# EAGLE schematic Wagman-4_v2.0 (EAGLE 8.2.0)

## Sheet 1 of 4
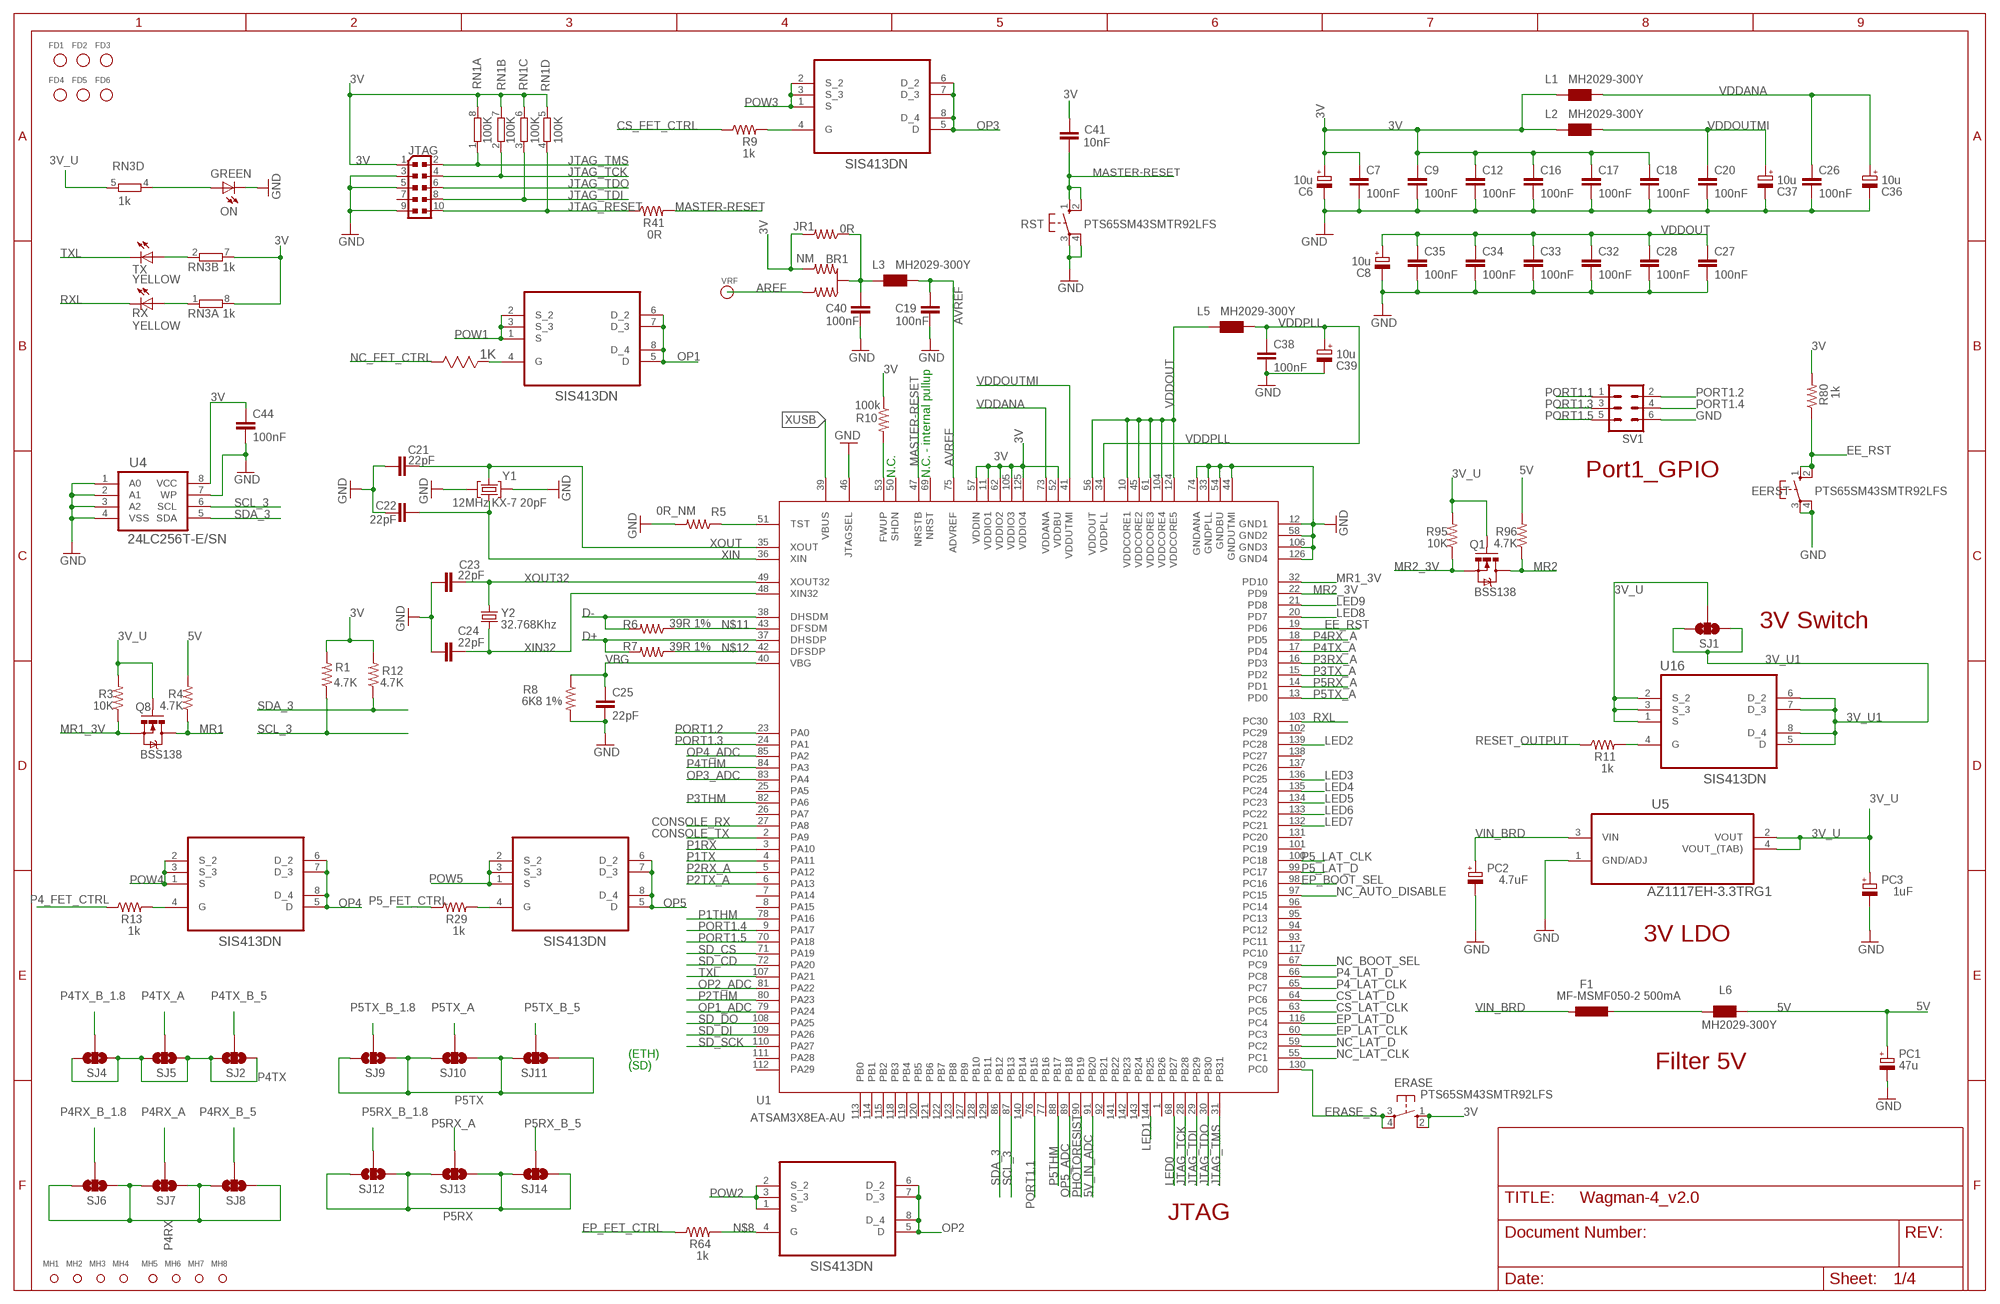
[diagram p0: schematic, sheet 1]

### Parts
BR1  NM  J0402  [J0402]
C6  10u  CPOL-EUSMCB  [SMC_B]
C7  100nF  CAP0805  [0805]
C8  10u  CPOL-EUSMCB  [SMC_B]
C9  100nF  CAP0805  [0805]
C12  100nF  CAP0805  [0805]
C16  100nF  CAP0805  [0805]
C17  100nF  CAP0805  [0805]
C18  100nF  CAP0805  [0805]
C19  100nF  CAP0805  [0805]
C20  100nF  CAP0805  [0805]
C21  22pF  CAP0805  [0805]
C22  22pF  CAP0805  [0805]
C23  22pF  CAP0805  [0805]
C24  22pF  CAP0805  [0805]
C25  22pF  CAP0805  [0805]
C26  100nF  CAP0805  [0805]
C27  100nF  CAP0805  [0805]
C28  100nF  CAP0805  [0805]
C32  100nF  CAP0805  [0805]
C33  100nF  CAP0805  [0805]
C34  100nF  CAP0805  [0805]
C35  100nF  CAP0805  [0805]
C36  10u  CPOL-EUSMCB  [SMC_B]
C37  10u  CPOL-EUSMCB  [SMC_B]
C38  100nF  CAP0805  [0805]
C39  10u  CPOL-EUSMCB  [SMC_B]
C40  100nF  CAP0805  [0805]
C41  10nF  CAP0805  [0805]
C44  100nF  CAP0805  [0805]
EERST  PTS65SM43SMTR92LFS  [TACT_SPST_SMD_6X6]
ERASE  PTS65SM43SMTR92LFS  [TACT_SPST_SMD_6X6]
F1  MF-MSMF050-2 500mA  L-EUL1812  [L1812]
FD1  FIDUCIAL-1MM  [FD-1MM]
FD2  FIDUCIAL-1MM  [FD-1MM]
FD3  FIDUCIAL-1MM  [FD-1MM]
FD4  FIDUCIAL-1MM  [FD-1MM]
FD5  FIDUCIAL-1MM  [FD-1MM]
FD6  FIDUCIAL-1MM  [FD-1MM]
JR1  0R  RESISTOR0805-RES  [0805]
JTAG  PINHEAD_PINHD-2X5PASSO127  [PINHEAD_2X05_127]
L1  MH2029-300Y  WE-CBF_0805  [0805]
L2  MH2029-300Y  WE-CBF_0805  [0805]
L3  MH2029-300Y  WE-CBF_0805  [0805]
L5  MH2029-300Y  WE-CBF_0805  [0805]
L6  MH2029-300Y  WE-CBF_0805  [0805]
MH1  MH-3.964  [MH3.964]
MH2  MH-3.964  [MH3.964]
MH3  MH-3.964  [MH3.964]
MH4  MH-3.964  [MH3.964]
MH5  MH-3.964  [MH3.964]
MH6  MH-3.964  [MH3.964]
MH7  MH-3.964  [MH3.964]
MH8  MH-3.964  [MH3.964]
ON  GREEN  LEDCHIPLED_0805  [CHIPLED_0805]
PC1  47u  CPOL-EUD  [PANASONIC_D]
PC2  4.7uF  CPOL-EUD  [PANASONIC_D]
PC3  1uF  CPOL-EUD  [PANASONIC_D]
Q1  BSS138  MOSFET-NCHANNELSMD  [SOT23-3]
Q8  BSS138  MOSFET-NCHANNELSMD  [SOT23-3]
R1  4.7K  RESISTOR0805-RES  [0805]
R3  10K  RESISTOR0805-RES  [0805]
R4  4.7K  RESISTOR0805-RES  [0805]
R5  0R_NM  RESISTOR0805-RES  [0805]
R6  39R 1%  RESISTOR0805-RES  [0805]
R7  39R 1%  RESISTOR0805-RES  [0805]
R8  6K8 1%  RESISTOR0805-RES  [0805]
R9  1k  RESISTOR0805-RES  [0805]
R10  100k  RESISTOR0805-RES  [0805]
R11  1k  RESISTOR0805-RES  [0805]
R12  4.7K  RESISTOR0805-RES  [0805]
R13  1k  RESISTOR0805-RES  [0805]
R29  1k  RESISTOR0805-RES  [0805]
R30  1K  CRM0805-FW-R050ELF  [0805]
R41  0R  RESISTOR0805-RES  [0805]
R64  1k  RESISTOR0805-RES  [0805]
R80  1k  RESISTOR0805-RES  [0805]
R95  10K  RESISTOR0805-RES  [0805]
R96  4.7K  RESISTOR0805-RES  [0805]
RN1  100K  4R-NCAT16  [CAT16]
RN3  1k  4R-NCAT16  [CAT16]
RST  PTS65SM43SMTR92LFS  [TACT_SPST_SMD_6X6]
RX  YELLOW  LEDCHIPLED_0805  [CHIPLED_0805]
SJ1  SOLDERJUMPER_2WAYPASTE1&2&3  [SJ_3_PASTE1&2&3]
SJ2  SOLDERJUMPER_2WAYPASTE1&2&3  [SJ_3_PASTE1&2&3]
SJ4  SOLDERJUMPER_2WAYPASTE1&2&3  [SJ_3_PASTE1&2&3]
SJ5  SOLDERJUMPER_2WAYPASTE1&2&3  [SJ_3_PASTE1&2&3]
SJ6  SOLDERJUMPER_2WAYPASTE1&2&3  [SJ_3_PASTE1&2&3]
SJ7  SOLDERJUMPER_2WAYPASTE1&2&3  [SJ_3_PASTE1&2&3]
SJ8  SOLDERJUMPER_2WAYPASTE1&2&3  [SJ_3_PASTE1&2&3]
SJ9  SOLDERJUMPER_2WAYPASTE1&2&3  [SJ_3_PASTE1&2&3]
SJ10  SOLDERJUMPER_2WAYPASTE1&2&3  [SJ_3_PASTE1&2&3]
SJ11  SOLDERJUMPER_2WAYPASTE1&2&3  [SJ_3_PASTE1&2&3]
SJ12  SOLDERJUMPER_2WAYPASTE1&2&3  [SJ_3_PASTE1&2&3]
SJ13  SOLDERJUMPER_2WAYPASTE1&2&3  [SJ_3_PASTE1&2&3]
SJ14  SOLDERJUMPER_2WAYPASTE1&2&3  [SJ_3_PASTE1&2&3]
SV1  MA03-2  [MA03-2]
TX  YELLOW  LEDCHIPLED_0805  [CHIPLED_0805]
U1  ATSAM3X8EA-AU  ATSAM3X/AAU  [LQFP144]
U3  SIS413DN  [SIS413]
U4  24LC256T-E/SN  [SOIC8]
U5  AZ1117EH-3.3TRG1  [SOT230P700X180-4N]
U6  SIS413DN  [SIS413]
U7  SIS413DN  [SIS413]
U8  SIS413DN  [SIS413]
U9  SIS413DN  [SIS413]
U16  SIS413DN  [SIS413]
VRF  FIDUCIAL-1MM  [FD-1MM]
Y1  12MHz KX-7 20pF  CRYSTAL-3.2-2.5  [CRYSTAL-3.2-2.5]
Y2  32.768Khz  RESONATOR_EPSON_FC_145  [RESONATOR_EPSON_FC_145]

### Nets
3V: BR1.3 C6.+ C7.1 C9.1 C12.1 C16.1 C17.1 C18.1 C41.1 C44.1 ERASE.1 ERASE.2 JR1.2 JTAG.1 L1.1 L2.1 R1.2 R10.1 R12.2 R80.2 RN1.5 RN1.6 RN1.7 RN1.8 RN3.7 RN3.8 U1.11(VDDIO1) U1.52(VDDBU) U1.57(VDDIN) U1.62(VDDIO2) U1.105(VDDIO3) U1.125(VDDIO4) U4.8(VCC) ; also sheet 2,3,4
3V_U: PC3.+ Q1.1(G) Q8.1(G) R3.2 R95.2 RN3.5 SJ1.2 U5.2(VOUT) U5.4(VOUT_(TAB)) U16.1(S) U16.2(S_2) U16.3(S_3) ; also sheet 2,3,4
3V_U1: SJ1.1 SJ1.3 U16.5(D) U16.6(D_2) U16.7(D_3) U16.8(D_4) ; also sheet 3
5V: L6.1 PC1.+ R4.2 R96.2 ; also sheet 2,3,4
5V_IN_ADC: U1.91(PB20) ; also sheet 4
AREF: BR1.1 VRF.1
AVREF: C19.1 L3.2 U1.75(ADVREF)
AVREFL: BR1.2(C) C40.1 JR1.1 L3.1
CONSOLE_RX: U1.27(PA8) ; also sheet 4
CONSOLE_TX: U1.2(PA9) ; also sheet 4
CS_FET_CTRL: R9.1 ; also sheet 4
CS_LAT_CLK: U1.63(PC5) ; also sheet 4
CS_LAT_D: U1.64(PC6) ; also sheet 4
D+: R7.2 U1.37(DHSDP) ; also sheet 2
D-: R6.2 U1.38(DHSDM) ; also sheet 2
EE_RST: EERST.1 EERST.2 R80.1 U1.19(PD6)
EP_BOOT_SEL: U1.98(PC16) ; also sheet 2
EP_FET_CTRL: R64.1 ; also sheet 4
EP_LAT_CLK: U1.60(PC3) ; also sheet 4
EP_LAT_D: U1.116(PC4) ; also sheet 4
ERASE_S: ERASE.3 ERASE.4 U1.130(PC0) ; also sheet 2,4
GND: C6.- C7.2 C8.- C9.2 C12.2 C16.2 C17.2 C18.2 C19.2 C20.2 C21.1 C22.2 C23.2 C24.2 C25.2 C26.2 C27.2 C28.2 C32.2 C33.2 C34.2 C35.2 C36.- C37.- C38.2 C39.- C40.2 C44.2 EERST.3 EERST.4 JTAG.3 JTAG.5 JTAG.9 ON.C PC1.- PC2.- PC3.- R5.2 R8.2 RST.3 RST.4 SV1.6 U1.12(GND1) U1.33(GNDPLL) U1.44(GNDUTMI) U1.46(JTAGSEL) U1.54(GNDBU) U1.58(GND2) U1.74(GNDANA) U1.106(GND3) U1.126(GND4) U4.1(A0) U4.2(A1) U4.3(A2) U4.4(VSS) U4.7(WP) U5.1(GND/ADJ) Y1.2(GND) Y1.4(GND) ; also sheet 2,3,4
JTAG_RESET: JTAG.10 R41.1 RN1.4
JTAG_TCK: JTAG.4 RN1.2 U1.28(PB28)
JTAG_TDI: JTAG.8 RN1.3 U1.29(PB29)
JTAG_TDO: JTAG.6 U1.30(PB30)
JTAG_TMS: JTAG.2 RN1.1 U1.31(PB31)
LED0: U1.68(PB27) ; also sheet 2
LED1: U1.144(PB25) ; also sheet 2
LED2: U1.139(PC28) ; also sheet 2
LED3: U1.136(PC25) ; also sheet 2
LED4: U1.135(PC24) ; also sheet 2
LED5: U1.134(PC23) ; also sheet 2
LED6: U1.133(PC22) ; also sheet 2
LED7: U1.132(PC21) ; also sheet 2
LED8: U1.20(PD7) ; also sheet 2
LED9: U1.21(PD8) ; also sheet 2
MASTER-RESET: C41.2 R41.2 RST.1 RST.2 U1.47(NRSTB) ; also sheet 2,4
MR1: Q8.3(D) R4.1 ; also sheet 3
MR1_3V: Q8.2(S) R3.1 U1.32(PD10)
MR2: Q1.3(D) R96.1 ; also sheet 3
MR2_3V: Q1.2(S) R95.1 U1.22(PD9)
N$1: ON.A RN3.4
N$5: R5.1 U1.51(TST)
N$7: R10.2 U1.53(FWUP)
N$8: R64.2 U6.4(G)
N$9: F1.1 L6.2
N$11: R6.1 U1.43(DFSDM)
N$12: R7.1 U1.42(DFSDP)
N$54: RN3.1 RX.A
N$55: RN3.2 TX.A
N$57: R11.2 U16.4(G)
N$77: R13.2 U3.4(G)
N$78: R9.2 U7.4(G)
N$79: R29.2 U8.4(G)
N$80: R30.2(R2) U9.4(G)
NC_AUTO_DISABLE: U1.97(PC15) ; also sheet 4
NC_BOOT_SEL: U1.67(PC9) ; also sheet 2
NC_FET_CTRL: R30.1(R1) ; also sheet 2
NC_LAT_CLK: U1.55(PC1) ; also sheet 4
NC_LAT_D: U1.59(PC2) ; also sheet 4
OP1: U9.5(D) U9.6(D_2) U9.7(D_3) U9.8(D_4) ; also sheet 2,3
OP1_ADC: U1.79(PA24) ; also sheet 4
OP2: U6.5(D) U6.6(D_2) U6.7(D_3) U6.8(D_4) ; also sheet 2,3
OP2_ADC: U1.81(PA22) ; also sheet 4
OP3: U7.5(D) U7.6(D_2) U7.7(D_3) U7.8(D_4) ; also sheet 2,3
OP3_ADC: U1.83(PA4) ; also sheet 4
OP4: U3.5(D) U3.6(D_2) U3.7(D_3) U3.8(D_4) ; also sheet 2,3
OP4_ADC: U1.85(PA2) ; also sheet 4
OP5: U8.5(D) U8.6(D_2) U8.7(D_3) U8.8(D_4) ; also sheet 2,3
OP5_ADC: U1.89(PB18) ; also sheet 4
P1RX: U1.3(PA10) ; also sheet 2
P1THM: U1.78(PA16) ; also sheet 2
P1TX: U1.4(PA11) ; also sheet 2
P2RX_A: U1.5(PA12) ; also sheet 3
P2THM: U1.80(PA23) ; also sheet 2
P2TX_A: U1.6(PA13) ; also sheet 3
P3RX_A: U1.16(PD3) ; also sheet 3
P3THM: U1.82(PA6) ; also sheet 2
P3TX_A: U1.15(PD2) ; also sheet 3
P4_FET_CTRL: R13.1 ; also sheet 4
P4_LAT_CLK: U1.65(PC7) ; also sheet 4
P4_LAT_D: U1.66(PC8) ; also sheet 4
P4RX: SJ6.1 SJ6.3 SJ7.1 SJ7.3 SJ8.1 SJ8.3 ; also sheet 2
P4RX_A: SJ7.2 U1.18(PD5) ; also sheet 3
P4RX_B_1.8: SJ6.2 ; also sheet 3
P4RX_B_5: SJ8.2 ; also sheet 3
P4THM: U1.84(PA3) ; also sheet 2
P4TX: SJ2.1 SJ2.3 SJ4.1 SJ4.3 SJ5.1 SJ5.3 ; also sheet 2
P4TX_A: SJ5.2 U1.17(PD4) ; also sheet 3
P4TX_B_1.8: SJ4.2 ; also sheet 3
P4TX_B_5: SJ2.2 ; also sheet 3
P5_FET_CTRL: R29.1 ; also sheet 4
P5_LAT_CLK: U1.100(PC18) ; also sheet 4
P5_LAT_D: U1.99(PC17) ; also sheet 4
P5RX: SJ12.1 SJ12.3 SJ13.1 SJ13.3 SJ14.1 SJ14.3 ; also sheet 2
P5RX_A: SJ13.2 U1.14(PD1) ; also sheet 3
P5RX_B_1.8: SJ12.2 ; also sheet 3
P5RX_B_5: SJ14.2 ; also sheet 3
P5THM: U1.88(PB17) ; also sheet 2
P5TX: SJ9.1 SJ9.3 SJ10.1 SJ10.3 SJ11.1 SJ11.3 ; also sheet 2
P5TX_A: SJ10.2 U1.13(PD0) ; also sheet 3
P5TX_B_1.8: SJ9.2 ; also sheet 3
P5TX_B_5: SJ11.2 ; also sheet 3
PHOTORESIST: U1.90(PB19) ; also sheet 2
PORT1.1: SV1.1 U1.76(PB15)
PORT1.2: SV1.2 U1.23(PA0)
PORT1.3: SV1.3 U1.24(PA1)
PORT1.4: SV1.4 U1.9(PA17)
PORT1.5: SV1.5 U1.70(PA18)
POW1: U9.1(S) U9.2(S_2) U9.3(S_3) ; also sheet 3,4
POW2: U6.1(S) U6.2(S_2) U6.3(S_3) ; also sheet 3,4
POW3: U7.1(S) U7.2(S_2) U7.3(S_3) ; also sheet 3,4
POW4: U3.1(S) U3.2(S_2) U3.3(S_3) ; also sheet 3,4
POW5: U8.1(S) U8.2(S_2) U8.3(S_3) ; also sheet 3,4
RESET_OUTPUT: R11.1 ; also sheet 3
RXL: RX.C U1.103(PC30)
SCL_3: R1.1 U1.87(PB13) U4.6(SCL) ; also sheet 2,3,4
SD_CD: U1.72(PA20) ; also sheet 4
SD_CS: U1.71(PA19) ; also sheet 4
SD_DI: U1.109(PA26) ; also sheet 4
SD_DO: U1.108(PA25) ; also sheet 4
SD_SCK: U1.110(PA27) ; also sheet 4
SDA_3: R12.1 U1.86(PB12) U4.5(SDA) ; also sheet 2,3,4
TXL: TX.C U1.107(PA21)
VBG: C25.1 R8.1 U1.40(VBG)
VDDANA: C26.1 C36.+ L1.2 U1.73(VDDANA)
VDDOUT: C8.+ C27.1 C28.1 C32.1 C33.1 C34.1 C35.1 L5.1 U1.10(VDDCORE1) U1.45(VDDCORE2) U1.56(VDDOUT) U1.61(VDDCORE3) U1.104(VDDCORE4) U1.124(VDDCORE5)
VDDOUTMI: C20.1 C37.+ L2.2 U1.41(VDDUTMI)
VDDPLL: C38.1 C39.+ L5.2 U1.34(VDDPLL)
VIN_BRD: F1.2 PC2.+ U5.3(VIN) ; also sheet 3,4
XIN: C22.1 U1.36(XIN) Y1.1(C1)
XIN32: C24.1 U1.48(XIN32) Y2.P$2
XOUT: C21.2 U1.35(XOUT) Y1.3(C2)
XOUT32: C23.1 U1.49(XOUT32) Y2.P$1
XUSB: U1.39(VBUS) ; also sheet 2
Unconnected: FD1.1 FD2.1 FD3.1 FD4.1 FD5.1 FD6.1 JTAG.7 MH1.1 MH2.1 MH3.1 MH4.1 MH5.1 MH6.1 MH7.1 MH8.1 RN3.3 RN3.6 U1.1(PB26) U1.7(PA14) U1.8(PA15) U1.25(PA5) U1.26(PA7) U1.50(SHDN) U1.69(NRST) U1.77(PB16) U1.92(PB21) U1.93(PC11) U1.94(PC12) U1.95(PC13) U1.96(PC14) U1.101(PC19) U1.102(PC29) U1.111(PA28) U1.112(PA29) U1.113(PB0) U1.114(PB1) U1.115(PB2) U1.117(PC10) U1.118(PB3) U1.119(PB4) U1.120(PB5) U1.121(PB6) U1.122(PB7) U1.123(PB8) U1.127(PB9) U1.128(PB10) U1.129(PB11) U1.131(PC20) U1.137(PC26) U1.138(PC27) U1.140(PB14) U1.141(PB22) U1.142(PB23) U1.143(PB24)

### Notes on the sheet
- N.C. | N.C. - internal pullup | Port1_GPIO
- 3V Switch
- 3V LDO
- (ETH)
- (SD) | Filter 5V
- JTAG

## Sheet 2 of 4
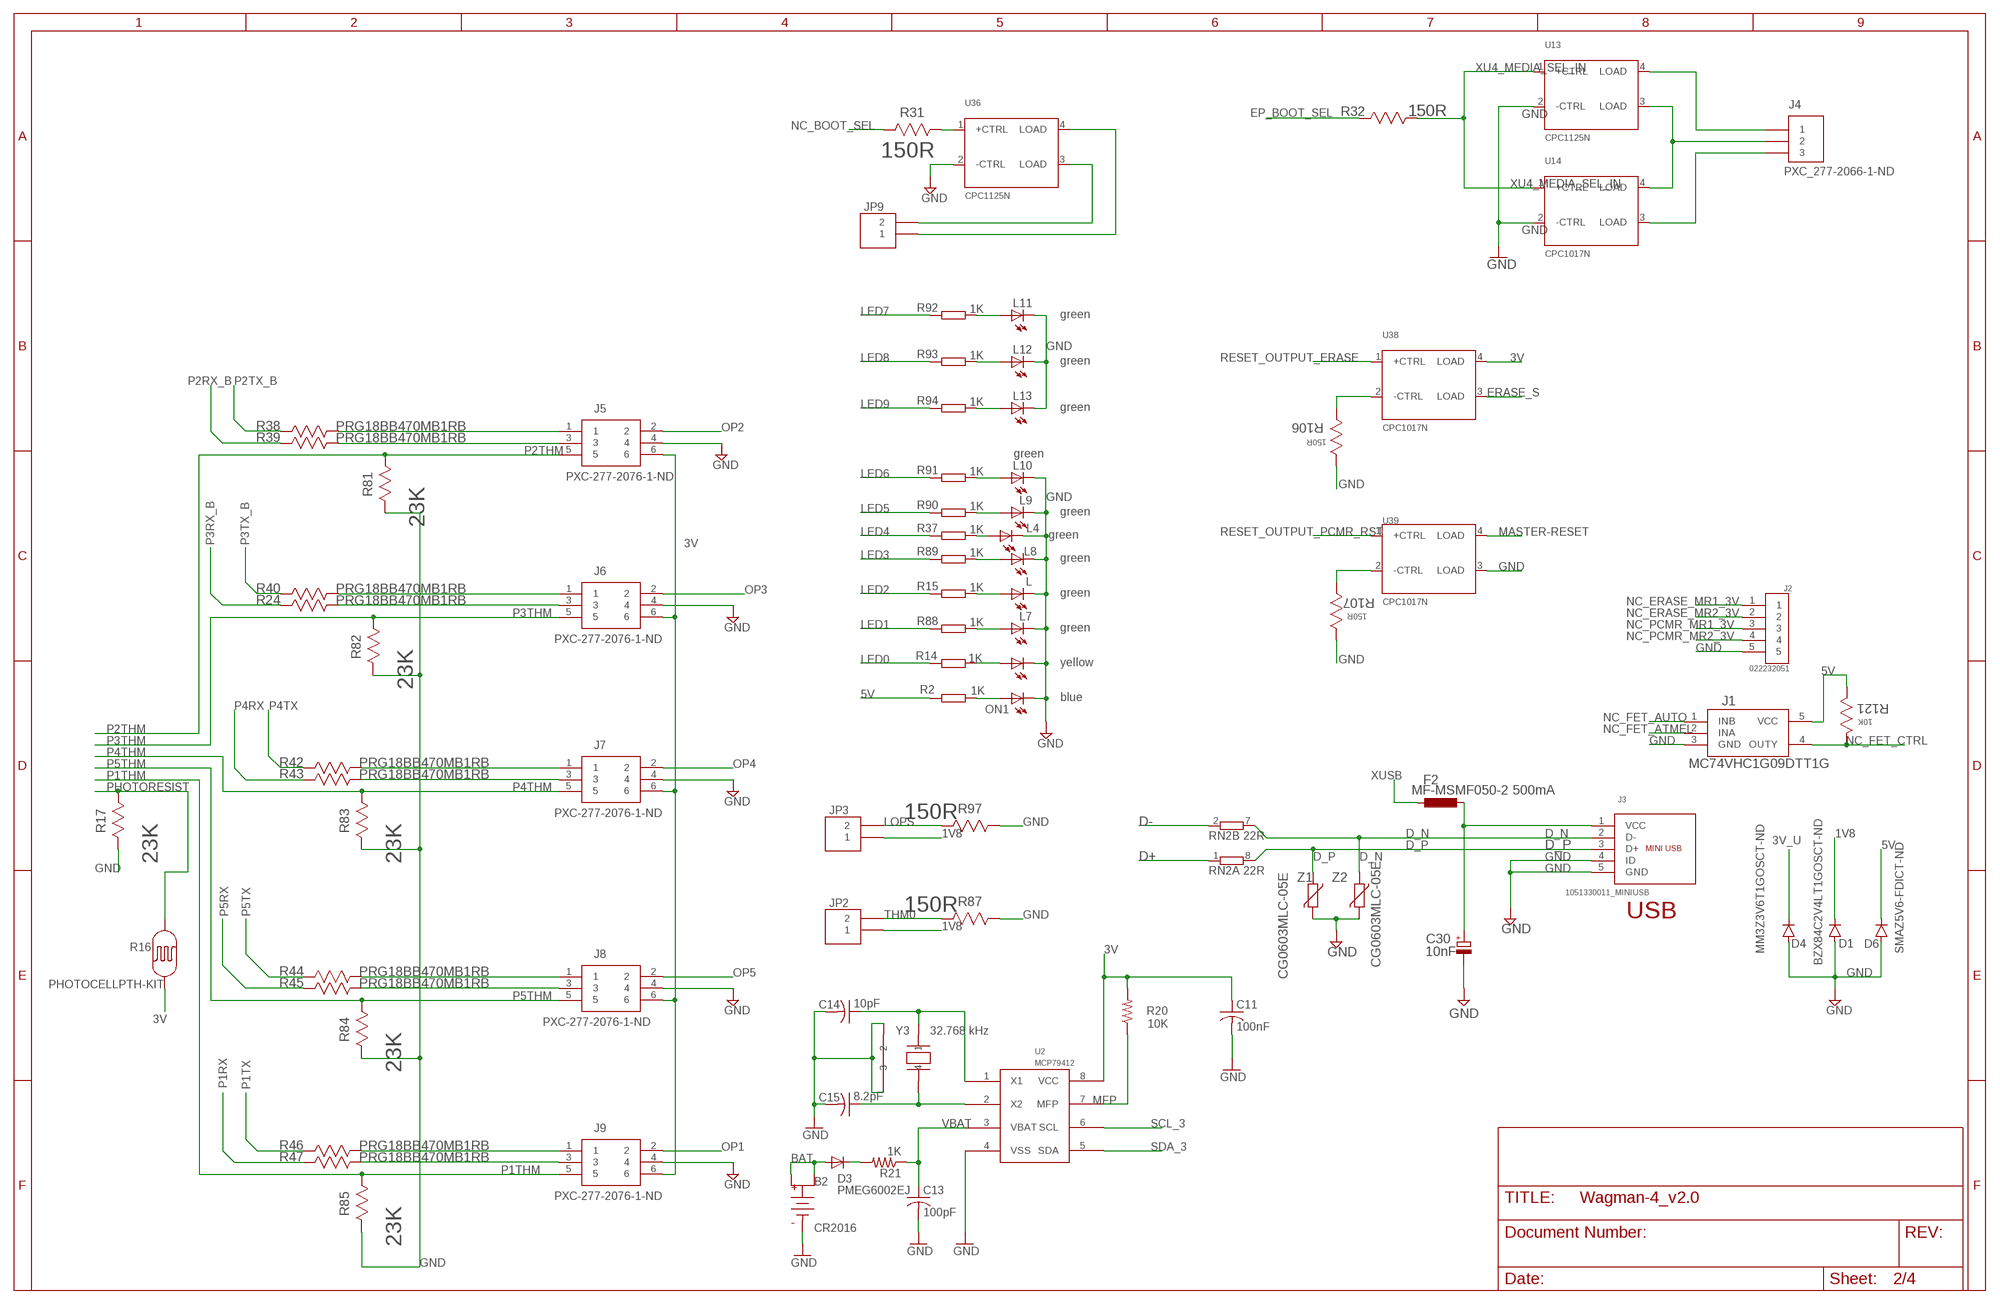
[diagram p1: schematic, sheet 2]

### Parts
B2  CR2016  COIN-CELL-2016-SMT  [BAT-HLD-002-SMT]
C11  100nF  C-USM0805  [M0805]
C13  100pF  C-USM0805  [M0805]
C14  10pF  C-USM0805  [M0805]
C15  8.2pF  C-USM0805  [M0805]
C30  10nF  CPOL-EUSMCB  [SMC_B]
D1  BZX84C2V4LT1GOSCT-ND  DIODESOT23  [SOT23-3]
D3  PMEG6002EJ  DIODESOD-323F  [SOD-323F]
D4  MM3Z3V6T1GOSCT-ND  DIODEBAS16  [SOD-323]
D6  SMAZ5V6-FDICT-ND  DIODESMA  [SMA-DIODE]
F2  MF-MSMF050-2 500mA  L-EUL1812  [L1812]
J1  MC74VHC1G09DTT1G  [TSOP-5]
J2  022232051  [01X05_P2.54_RELIMATE]
J3  1051330011_MINIUSB  [1051330011_MINIUSB_VERTICAL]
J4  PXC_277-2066-1-ND  [3PIN-PTSM-RA-2.5MM]
J5  PXC-277-2076-1-ND  [6PIN-PTSM-2.5MM]
J6  PXC-277-2076-1-ND  [6PIN-PTSM-2.5MM]
J7  PXC-277-2076-1-ND  [6PIN-PTSM-2.5MM]
J8  PXC-277-2076-1-ND  [6PIN-PTSM-2.5MM]
J9  PXC-277-2076-1-ND  [6PIN-PTSM-2.5MM]
JP2  CONN_2PINCONN_2PIN_P2.54MM  [CONN_2PIN_P2.54MM]
JP3  CONN_2PINCONN_2PIN_P2.54MM  [CONN_2PIN_P2.54MM]
JP9  CONN_2PINCONN_2PIN_P2.54MM  [CONN_2PIN_P2.54MM]
L  green  LEDCHIPLED_0805  [CHIPLED_0805]
L4  green  LEDCHIPLED_0805  [CHIPLED_0805]
L7  green  LEDCHIPLED_0805  [CHIPLED_0805]
L8  green  LEDCHIPLED_0805  [CHIPLED_0805]
L9  green  LEDCHIPLED_0805  [CHIPLED_0805]
L10  green  LEDCHIPLED_0805  [CHIPLED_0805]
L11  green  LEDCHIPLED_0805  [CHIPLED_0805]
L12  green  LEDCHIPLED_0805  [CHIPLED_0805]
L13  green  LEDCHIPLED_0805  [CHIPLED_0805]
ON1  blue  LEDCHIPLED_0805  [CHIPLED_0805]
R2  1K  R-EU_R0402  [R0402]
R14  1K  R-EU_R0402  [R0402]
R15  1K  R-EU_R0402  [R0402]
R16  PHOTOCELLPTH-KIT  [PHOTOCELL-KIT]
R17  23K  CRM0805-FW-R050ELF  [RESC2013X65N]
R20  10K  R-US_M0805  [M0805]
R21  1K  R-US_M0805  [M0805]
R24  PRG18BB470MB1RB  PTC-SMD  [PTC-0603]
R31  150R  CRM0805-FW-R050ELF  [RESC2013X65N]
R32  150R  CRM0805-FW-R050ELF  [RESC2013X65N]
R37  1K  R-EU_R0402  [R0402]
R38  PRG18BB470MB1RB  PTC-SMD  [PTC-0603]
R39  PRG18BB470MB1RB  PTC-SMD  [PTC-0603]
R40  PRG18BB470MB1RB  PTC-SMD  [PTC-0603]
R42  PRG18BB470MB1RB  PTC-SMD  [PTC-0603]
R43  PRG18BB470MB1RB  PTC-SMD  [PTC-0603]
R44  PRG18BB470MB1RB  PTC-SMD  [PTC-0603]
R45  PRG18BB470MB1RB  PTC-SMD  [PTC-0603]
R46  PRG18BB470MB1RB  PTC-SMD  [PTC-0603]
R47  PRG18BB470MB1RB  PTC-SMD  [PTC-0603]
R81  23K  CRM0805-FW-R050ELF  [RESC2013X65N]
R82  23K  CRM0805-FW-R050ELF  [RESC2013X65N]
R83  23K  CRM0805-FW-R050ELF  [RESC2013X65N]
R84  23K  CRM0805-FW-R050ELF  [RESC2013X65N]
R85  23K  CRM0805-FW-R050ELF  [RESC2013X65N]
R87  150R  CRM0805-FW-R050ELF  [RESC2013X65N]
R88  1K  R-EU_R0402  [R0402]
R89  1K  R-EU_R0402  [R0402]
R90  1K  R-EU_R0402  [R0402]
R91  1K  R-EU_R0402  [R0402]
R92  1K  R-EU_R0402  [R0402]
R93  1K  R-EU_R0402  [R0402]
R94  1K  R-EU_R0402  [R0402]
R97  150R  CRM0805-FW-R050ELF  [RESC2013X65N]
R106  150R  CRM0805-FW-R050ELF  [RESC2013X65N]
R107  150R  CRM0805-FW-R050ELF  [RESC2013X65N]
R121  10K  CRM0805-FW-R050ELF  [RESC2013X65N]
RN2  22R  4R-NCAY16  [CAY16]
TX1  yellow  LEDCHIPLED_0805  [CHIPLED_0805]
U2  MCP79412  MCP7941X-SOIC-8  [SO08]
U13  CPC1125N  [SOP-4]
U14  CPC1017N  CPC1125N  [SOP-4]
U36  CPC1125N  [SOP-4]
U38  CPC1017N  CPC1125N  [SOP-4]
U39  CPC1017N  CPC1125N  [SOP-4]
Y3  32.768 kHz  CRYSTAL-CITIZEN-CM2XXC  [CRYSTAL-CITIZEN-CM2XXC]
Z1  CG0603MLC-05E  VARISTORCN0603  [CT/CN0603]
Z2  CG0603MLC-05E  VARISTORCN0603  [CT/CN0603]

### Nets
1V8: D1.3(C) JP2.1 JP3.1 ; also sheet 3
3V: C11.1 J5.6 J6.6 J7.6 J8.6 J9.6 R16.1 R20.2 U2.8(VCC) U38.4(LOAD) ; also sheet 1,3,4
3V_U: D4.C ; also sheet 1,3,4
5V: D6.C J1.5(VCC) R2.1 R121.2(R2) ; also sheet 1,3,4
BAT: B2.POS1 B2.POS2 D3.A
D+: RN2.1 ; also sheet 1
D-: RN2.2 ; also sheet 1
D_N: J3.2(D-) RN2.7 Z2.1
D_P: J3.3(D+) RN2.8 Z1.1
EP_BOOT_SEL: R32.2(R2) ; also sheet 1
ERASE_S: U38.3(LOAD) ; also sheet 1,4
GND: B2.NEG(B-) C11.2 C13.2 C14.2 C15.2 C30.- D1.1(A) D4.A D6.A J1.3(GND) J2.5 J3.4(ID) J3.5(GND) J5.4 J6.4 J7.4 J8.4 J9.4 L4.C L7.C L8.C L9.C L10.C L11.C L12.C L13.C L.C ON1.C R17.2(R2) R81.2(R2) R82.2(R2) R83.2(R2) R84.2(R2) R85.2(R2) R87.1(R1) R97.1(R1) R106.2(R2) R107.2(R2) TX1.C U2.4(VSS) U13.2(-CTRL) U14.2(-CTRL) U36.2(-CTRL) U39.3(LOAD) Y3.P$2 Y3.P$3 Z1.2 Z2.2 ; also sheet 1,3,4
LED0: R14.1 ; also sheet 1
LED1: R88.1 ; also sheet 1
LED2: R15.1 ; also sheet 1
LED3: R89.1 ; also sheet 1
LED4: R37.1 ; also sheet 1
LED5: R90.1 ; also sheet 1
LED6: R91.1 ; also sheet 1
LED7: R92.1 ; also sheet 1
LED8: R93.1 ; also sheet 1
LED9: R94.1 ; also sheet 1
LOPS: JP3.2 R97.2(R2) ; also sheet 4
MASTER-RESET: U39.4(LOAD) ; also sheet 1,4
MFP: R20.1 U2.7(MFP)
N$3: L.A R15.2
N$4: R14.2 TX1.A
N$10: ON1.A R2.2
N$15: C15.1 U2.2(X2) Y3.P$4
N$16: JP9.2 U36.3(LOAD)
N$17: C14.1 U2.1(X1) Y3.P$1
N$21: D3.K R21.2
N$22: L7.A R88.2
N$23: JP9.1 U36.4(LOAD)
N$25: L4.A R37.2
N$29: J5.1 R38.1(R1)
N$31: J5.3 R39.1(R1)
N$32: J6.1 R40.1(R1)
N$33: J6.3 R24.1(R1)
N$34: J7.1 R42.1(R1)
N$35: J7.3 R43.1(R1)
N$36: J8.1 R44.1(R1)
N$37: J8.3 R45.1(R1)
N$38: J9.1 R46.1(R1)
N$39: J9.3 R47.1(R1)
N$40: R31.1(R1) U36.1(+CTRL)
N$42: J4.2 U13.3(LOAD) U14.4(LOAD)
N$43: J4.1 U13.4(LOAD)
N$44: J4.3 U14.3(LOAD)
N$68: L8.A R89.2
N$69: L9.A R90.2
N$70: L10.A R91.2
N$71: L11.A R92.2
N$72: L12.A R93.2
N$73: L13.A R94.2
N$82: R106.1(R1) U38.2(-CTRL)
N$83: R107.1(R1) U39.2(-CTRL)
NC_BOOT_SEL: R31.2(R2) ; also sheet 1
NC_ERASE_MR1_3V: J2.1 ; also sheet 3
NC_ERASE_MR2_3V: J2.2 ; also sheet 3
NC_FET_ATMEL: J1.2(INA) ; also sheet 4
NC_FET_AUTO: J1.1(INB) ; also sheet 4
NC_FET_CTRL: J1.4(OUTY) R121.1(R1) ; also sheet 1
NC_PCMR_MR1_3V: J2.3 ; also sheet 3
NC_PCMR_MR2_3V: J2.4 ; also sheet 3
OP1: J9.2 ; also sheet 1,3
OP2: J5.2 ; also sheet 1,3
OP3: J6.2 ; also sheet 1,3
OP4: J7.2 ; also sheet 1,3
OP5: J8.2 ; also sheet 1,3
P1RX: R47.2(R2) ; also sheet 1
P1THM: J9.5 R85.1(R1) ; also sheet 1
P1TX: R46.2(R2) ; also sheet 1
P2RX_B: R39.2(R2) ; also sheet 3
P2THM: J5.5 R81.1(R1) ; also sheet 1
P2TX_B: R38.2(R2) ; also sheet 3
P3RX_B: R24.2(R2) ; also sheet 3
P3THM: J6.5 R82.1(R1) ; also sheet 1
P3TX_B: R40.2(R2) ; also sheet 3
P4RX: R43.2(R2) ; also sheet 1
P4THM: J7.5 R83.1(R1) ; also sheet 1
P4TX: R42.2(R2) ; also sheet 1
P5RX: R45.2(R2) ; also sheet 1
P5THM: J8.5 R84.1(R1) ; also sheet 1
P5TX: R44.2(R2) ; also sheet 1
PHOTORESIST: R16.2 R17.1(R1) ; also sheet 1
RESET_OUTPUT_ERASE: U38.1(+CTRL) ; also sheet 3
RESET_OUTPUT_PCMR_RST: U39.1(+CTRL) ; also sheet 3
SCL_3: U2.6(SCL) ; also sheet 1,3,4
SDA_3: U2.5(SDA) ; also sheet 1,3,4
THM0: JP2.2 R87.2(R2) ; also sheet 4
VBAT: C13.1 R21.1 U2.3(VBAT)
VUSBD: C30.+ F2.1 J3.1(VCC)
XU4_MEDIA_SEL_IN: R32.1(R1) U13.1(+CTRL) U14.1(+CTRL)
XUSB: F2.2 ; also sheet 1
Unconnected: J3.6 J3.7 J3.8 J3.9 J3.10 J3.11 J3.12 J3.13 J3.14 RN2.3 RN2.4 RN2.5 RN2.6

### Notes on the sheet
- USB

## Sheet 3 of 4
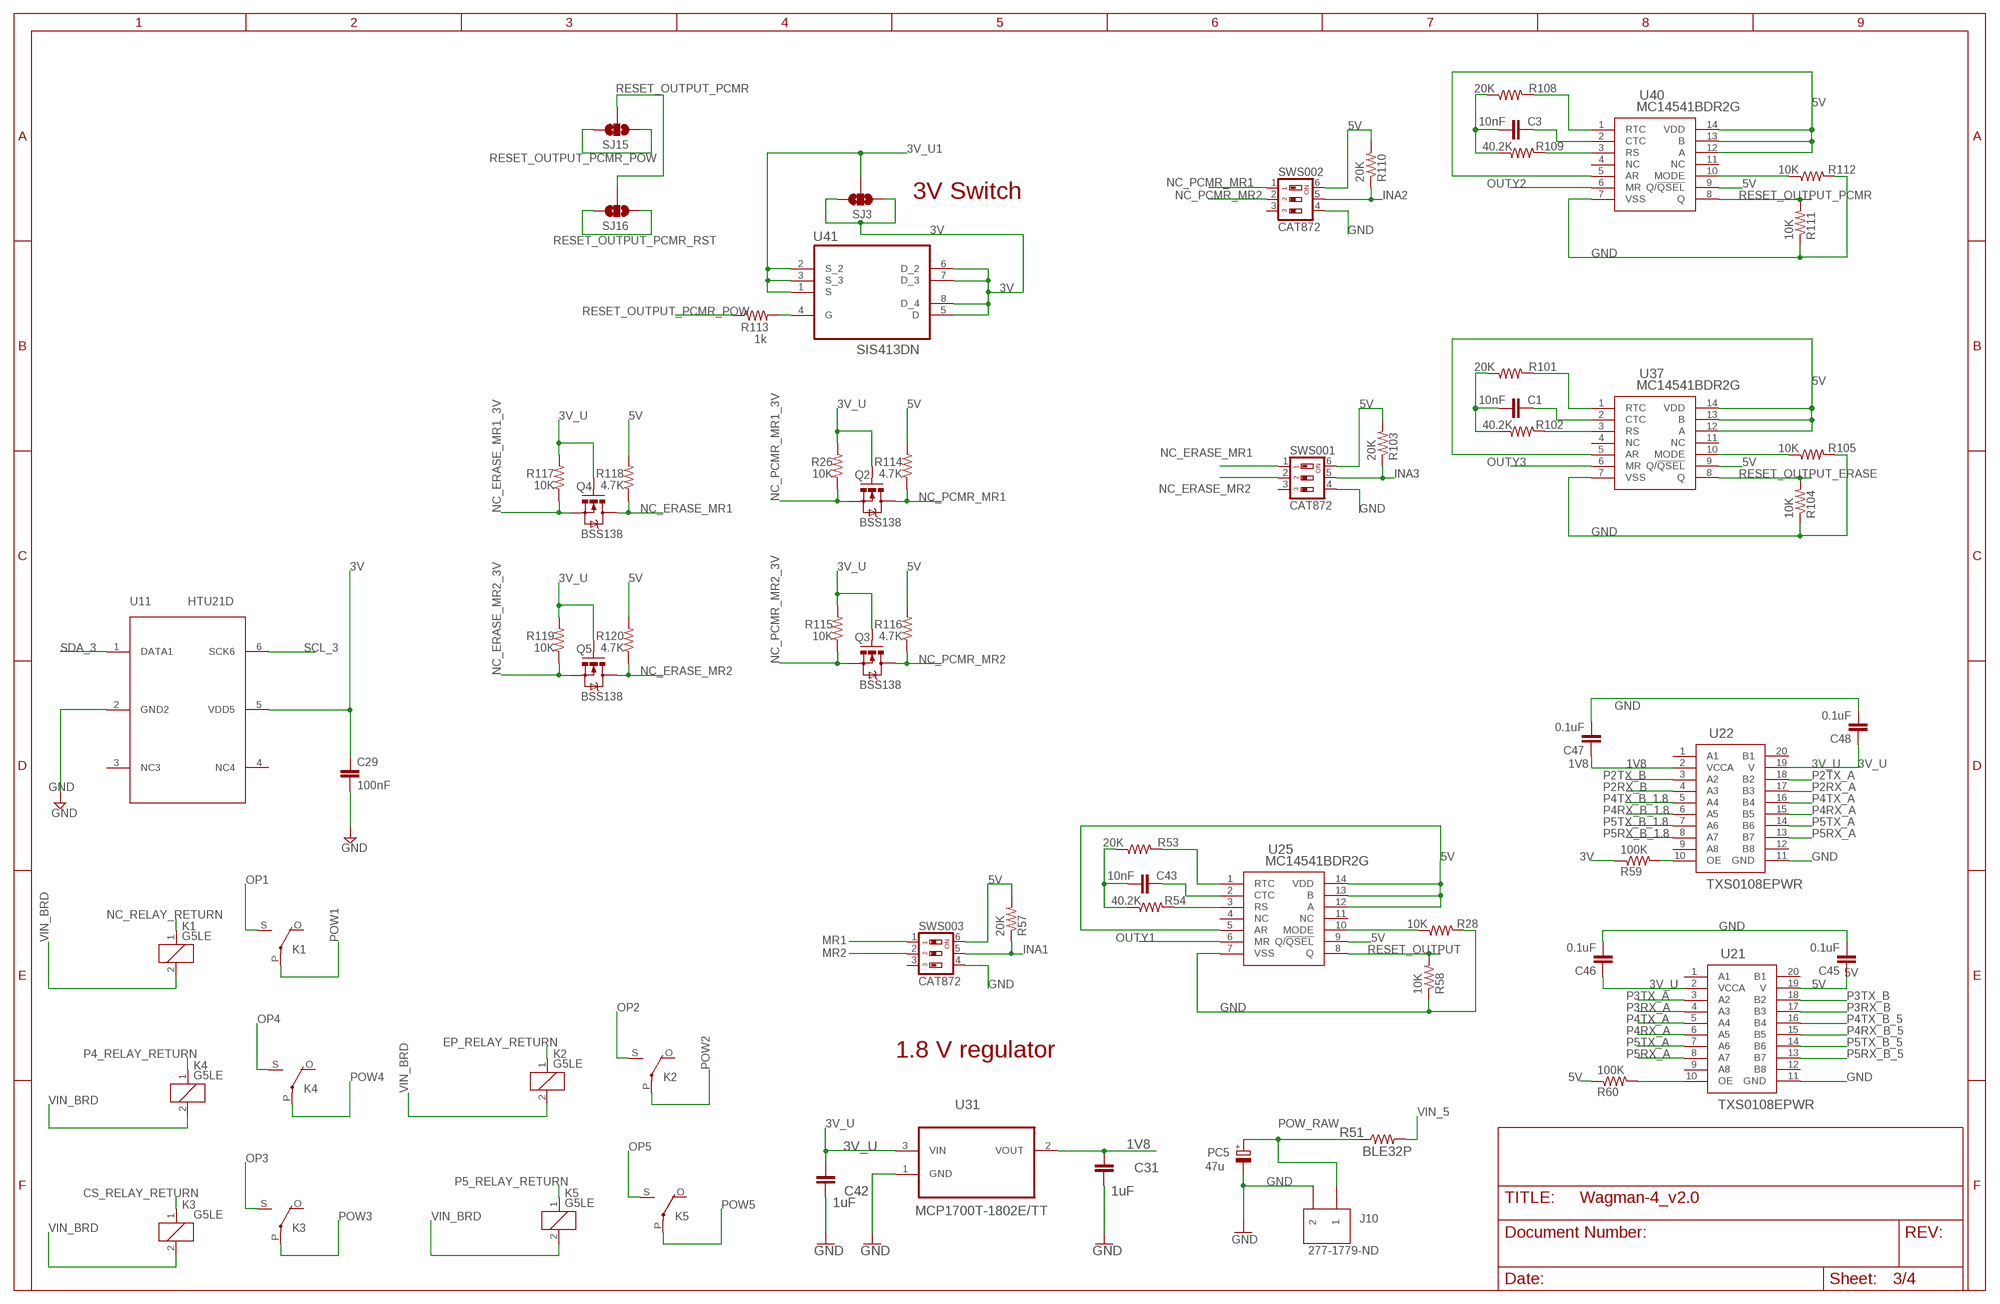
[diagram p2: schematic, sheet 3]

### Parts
C1  10nF  C-EUC0805  [C0805]
C3  10nF  C-EUC0805  [C0805]
C29  100nF  CAP0603-CAP  [0603-CAP]
C31  1uF  CAP0805  [0805]
C42  1uF  CAP0805  [0805]
C43  10nF  C-EUC0805  [C0805]
C45  0.1uF  C-EUC0805  [C0805]
C46  0.1uF  C-EUC0805  [C0805]
C47  0.1uF  C-EUC0805  [C0805]
C48  0.1uF  C-EUC0805  [C0805]
J10  277-1779-ND  TB2-3.5MM  [TB2-3.5MM]
K1  G5LE  [G5LE]
K2  G5LE  [G5LE]
K3  G5LE  [G5LE]
K4  G5LE  [G5LE]
K5  G5LE  [G5LE]
PC5  47u  CPOL-EUD  [PANASONIC_D]
Q2  BSS138  MOSFET-NCHANNELSMD  [SOT23-3]
Q3  BSS138  MOSFET-NCHANNELSMD  [SOT23-3]
Q4  BSS138  MOSFET-NCHANNELSMD  [SOT23-3]
Q5  BSS138  MOSFET-NCHANNELSMD  [SOT23-3]
R26  10K  RESISTOR0805-RES  [0805]
R28  10K  R-US_R0805  [R0805]
R51  BLE32P  R-US_R1210  [R1210]
R53  20K  R-US_R0805  [R0805]
R54  40.2K  R-US_R0805  [R0805]
R57  20K  R-US_R0805  [R0805]
R58  10K  R-US_R0805  [R0805]
R59  100K  R-US_R0805  [R0805]
R60  100K  R-US_R0805  [R0805]
R101  20K  R-US_R0805  [R0805]
R102  40.2K  R-US_R0805  [R0805]
R103  20K  R-US_R0805  [R0805]
R104  10K  R-US_R0805  [R0805]
R105  10K  R-US_R0805  [R0805]
R108  20K  R-US_R0805  [R0805]
R109  40.2K  R-US_R0805  [R0805]
R110  20K  R-US_R0805  [R0805]
R111  10K  R-US_R0805  [R0805]
R112  10K  R-US_R0805  [R0805]
R113  1k  RESISTOR0805-RES  [0805]
R114  4.7K  RESISTOR0805-RES  [0805]
R115  10K  RESISTOR0805-RES  [0805]
R116  4.7K  RESISTOR0805-RES  [0805]
R117  10K  RESISTOR0805-RES  [0805]
R118  4.7K  RESISTOR0805-RES  [0805]
R119  10K  RESISTOR0805-RES  [0805]
R120  4.7K  RESISTOR0805-RES  [0805]
SJ3  SOLDERJUMPER_2WAYPASTE1&2&3  [SJ_3_PASTE1&2&3]
SJ15  SOLDERJUMPER_2WAYPASTE1&2&3  [SJ_3_PASTE1&2&3]
SJ16  SOLDERJUMPER_2WAYPASTE1&2&3  [SJ_3_PASTE1&2&3]
SWS001  CAT872  [CAT872]
SWS002  CAT872  [CAT872]
SWS003  CAT872  [CAT872]
U11  HTU21D  [DD8-3X3MM]
U21  TXS0108EPWR  [PW20]
U22  TXS0108EPWR  [PW20]
U25  MC14541BDR2G  [SOIC14-3.9MM]
U31  MCP1700T-1802E/TT  [SOT95P237X112-3N]
U37  MC14541BDR2G  [SOIC14-3.9MM]
U40  MC14541BDR2G  [SOIC14-3.9MM]
U41  SIS413DN  [SIS413]

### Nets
1V8: C31.1 C47.1 U22.2(VCCA) U31.2(VOUT) ; also sheet 2
3V: C29.1 R59.1 SJ3.1 SJ3.3 U11.5(VDD5) U41.5(D) U41.6(D_2) U41.7(D_3) U41.8(D_4) ; also sheet 1,2,4
3V_U: C42.1 C46.1 C48.1 Q2.1(G) Q3.1(G) Q4.1(G) Q5.1(G) R26.2 R115.2 R117.2 R119.2 U21.2(VCCA) U22.19(V) U31.3(VIN) ; also sheet 1,2,4
3V_U1: SJ3.2 U41.1(S) U41.2(S_2) U41.3(S_3) ; also sheet 1
5V: C45.1 R57.2 R60.1 R103.2 R110.2 R114.2 R116.2 R118.2 R120.2 SWS001.6 SWS002.6 SWS003.6 U21.19(V) U25.5(AR) U25.9(Q/!QSEL) U25.12(A) U25.13(B) U25.14(VDD) U37.5(AR) U37.9(Q/!QSEL) U37.12(A) U37.13(B) U37.14(VDD) U40.5(AR) U40.9(Q/!QSEL) U40.12(A) U40.13(B) U40.14(VDD) ; also sheet 1,2,4
CS_RELAY_RETURN: K3.1 ; also sheet 4
EP_RELAY_RETURN: K2.1 ; also sheet 4
GND: C29.2 C31.2 C42.2 C45.2 C46.2 C47.2 C48.2 J10.P$2 PC5.- R28.2 R58.1 R104.1 R105.2 R111.1 R112.2 SWS001.4 SWS002.4 SWS003.4 U11.2(GND2) U21.11(GND) U22.11(GND) U25.7(VSS) U31.1(GND) U37.7(VSS) U40.7(VSS) ; also sheet 1,2,4
INA1: R57.1 SWS003.5 ; also sheet 4
INA2: R110.1 SWS002.5 ; also sheet 4
INA3: R103.1 SWS001.5 ; also sheet 4
MR1: SWS003.1 ; also sheet 1
MR2: SWS003.2 ; also sheet 1
N$2: R102.2 U37.3(RS)
N$13: R28.1 U25.10(MODE)
N$19: R60.2 U21.10(OE)
N$50: R54.2 U25.3(RS)
N$51: C43.1 U25.2(CTC)
N$52: R53.2 U25.1(RTC)
N$53: C43.2 R53.1 R54.1
N$56: R59.2 U22.10(OE)
N$74: C1.1 U37.2(CTC)
N$75: R101.2 U37.1(RTC)
N$76: C1.2 R101.1 R102.1
N$81: R105.1 U37.10(MODE)
N$84: R109.2 U40.3(RS)
N$85: C3.1 U40.2(CTC)
N$86: R108.2 U40.1(RTC)
N$87: C3.2 R108.1 R109.1
N$88: R112.1 U40.10(MODE)
N$89: R113.2 U41.4(G)
NC_ERASE_MR1: Q4.3(D) R118.1 SWS001.1
NC_ERASE_MR1_3V: Q4.2(S) R117.1 ; also sheet 2
NC_ERASE_MR2: Q5.3(D) R120.1 SWS001.2
NC_ERASE_MR2_3V: Q5.2(S) R119.1 ; also sheet 2
NC_PCMR_MR1: Q2.3(D) R114.1 SWS002.1
NC_PCMR_MR1_3V: Q2.2(S) R26.1 ; also sheet 2
NC_PCMR_MR2: Q3.3(D) R116.1 SWS002.2
NC_PCMR_MR2_3V: Q3.2(S) R115.1 ; also sheet 2
NC_RELAY_RETURN: K1.1 ; also sheet 4
OP1: K1.S(2:S) ; also sheet 1,2
OP2: K2.S(2:S) ; also sheet 1,2
OP3: K3.S(2:S) ; also sheet 1,2
OP4: K4.S(2:S) ; also sheet 1,2
OP5: K5.S(2:S) ; also sheet 1,2
OUTY1: U25.6(MR) ; also sheet 4
OUTY2: U40.6(MR) ; also sheet 4
OUTY3: U37.6(MR) ; also sheet 4
P2RX_A: U22.17(B3) ; also sheet 1
P2RX_B: U22.4(A3) ; also sheet 2
P2TX_A: U22.18(B2) ; also sheet 1
P2TX_B: U22.3(A2) ; also sheet 2
P3RX_A: U21.4(A3) ; also sheet 1
P3RX_B: U21.17(B3) ; also sheet 2
P3TX_A: U21.3(A2) ; also sheet 1
P3TX_B: U21.18(B2) ; also sheet 2
P4_RELAY_RETURN: K4.1 ; also sheet 4
P4RX_A: U21.6(A5) U22.15(B5) ; also sheet 1
P4RX_B_1.8: U22.6(A5) ; also sheet 1
P4RX_B_5: U21.15(B5) ; also sheet 1
P4TX_A: U21.5(A4) U22.16(B4) ; also sheet 1
P4TX_B_1.8: U22.5(A4) ; also sheet 1
P4TX_B_5: U21.16(B4) ; also sheet 1
P5_RELAY_RETURN: K5.1 ; also sheet 4
P5RX_A: U21.8(A7) U22.13(B7) ; also sheet 1
P5RX_B_1.8: U22.8(A7) ; also sheet 1
P5RX_B_5: U21.13(B7) ; also sheet 1
P5TX_A: U21.7(A6) U22.14(B6) ; also sheet 1
P5TX_B_1.8: U22.7(A6) ; also sheet 1
P5TX_B_5: U21.14(B6) ; also sheet 1
POW1: K1.P(2:P) ; also sheet 1,4
POW2: K2.P(2:P) ; also sheet 1,4
POW3: K3.P(2:P) ; also sheet 1,4
POW4: K4.P(2:P) ; also sheet 1,4
POW5: K5.P(2:P) ; also sheet 1,4
POW_RAW: J10.P$1 PC5.+ R51.1 ; also sheet 4
RESET_OUTPUT: R58.2 U25.8(Q) ; also sheet 1
RESET_OUTPUT_ERASE: R104.2 U37.8(Q) ; also sheet 2
RESET_OUTPUT_PCMR: R111.2 SJ15.2 SJ16.2 U40.8(Q)
RESET_OUTPUT_PCMR_POW: R113.1 SJ15.1 SJ15.3
RESET_OUTPUT_PCMR_RST: SJ16.1 SJ16.3 ; also sheet 2
SCL_3: U11.6(SCK6) ; also sheet 1,2,4
SDA_3: U11.1(DATA1) ; also sheet 1,2,4
VIN_5: R51.2 ; also sheet 4
VIN_BRD: K1.2 K2.2 K3.2 K4.2 K5.2 ; also sheet 1,4
Unconnected: K1.O(2:O) K2.O(2:O) K3.O(2:O) K4.O(2:O) K5.O(2:O) SWS001.3 SWS002.3 SWS003.3 U11.3(NC3) U11.4(NC4) U21.1(A1) U21.9(A8) U21.12(B8) U21.20(B1) U22.1(A1) U22.9(A8) U22.12(B8) U22.20(B1) U25.4(NC) U25.11(NC) U37.4(NC) U37.11(NC) U40.4(NC) U40.11(NC)

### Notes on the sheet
- 3V Switch
- 1.8 V regulator

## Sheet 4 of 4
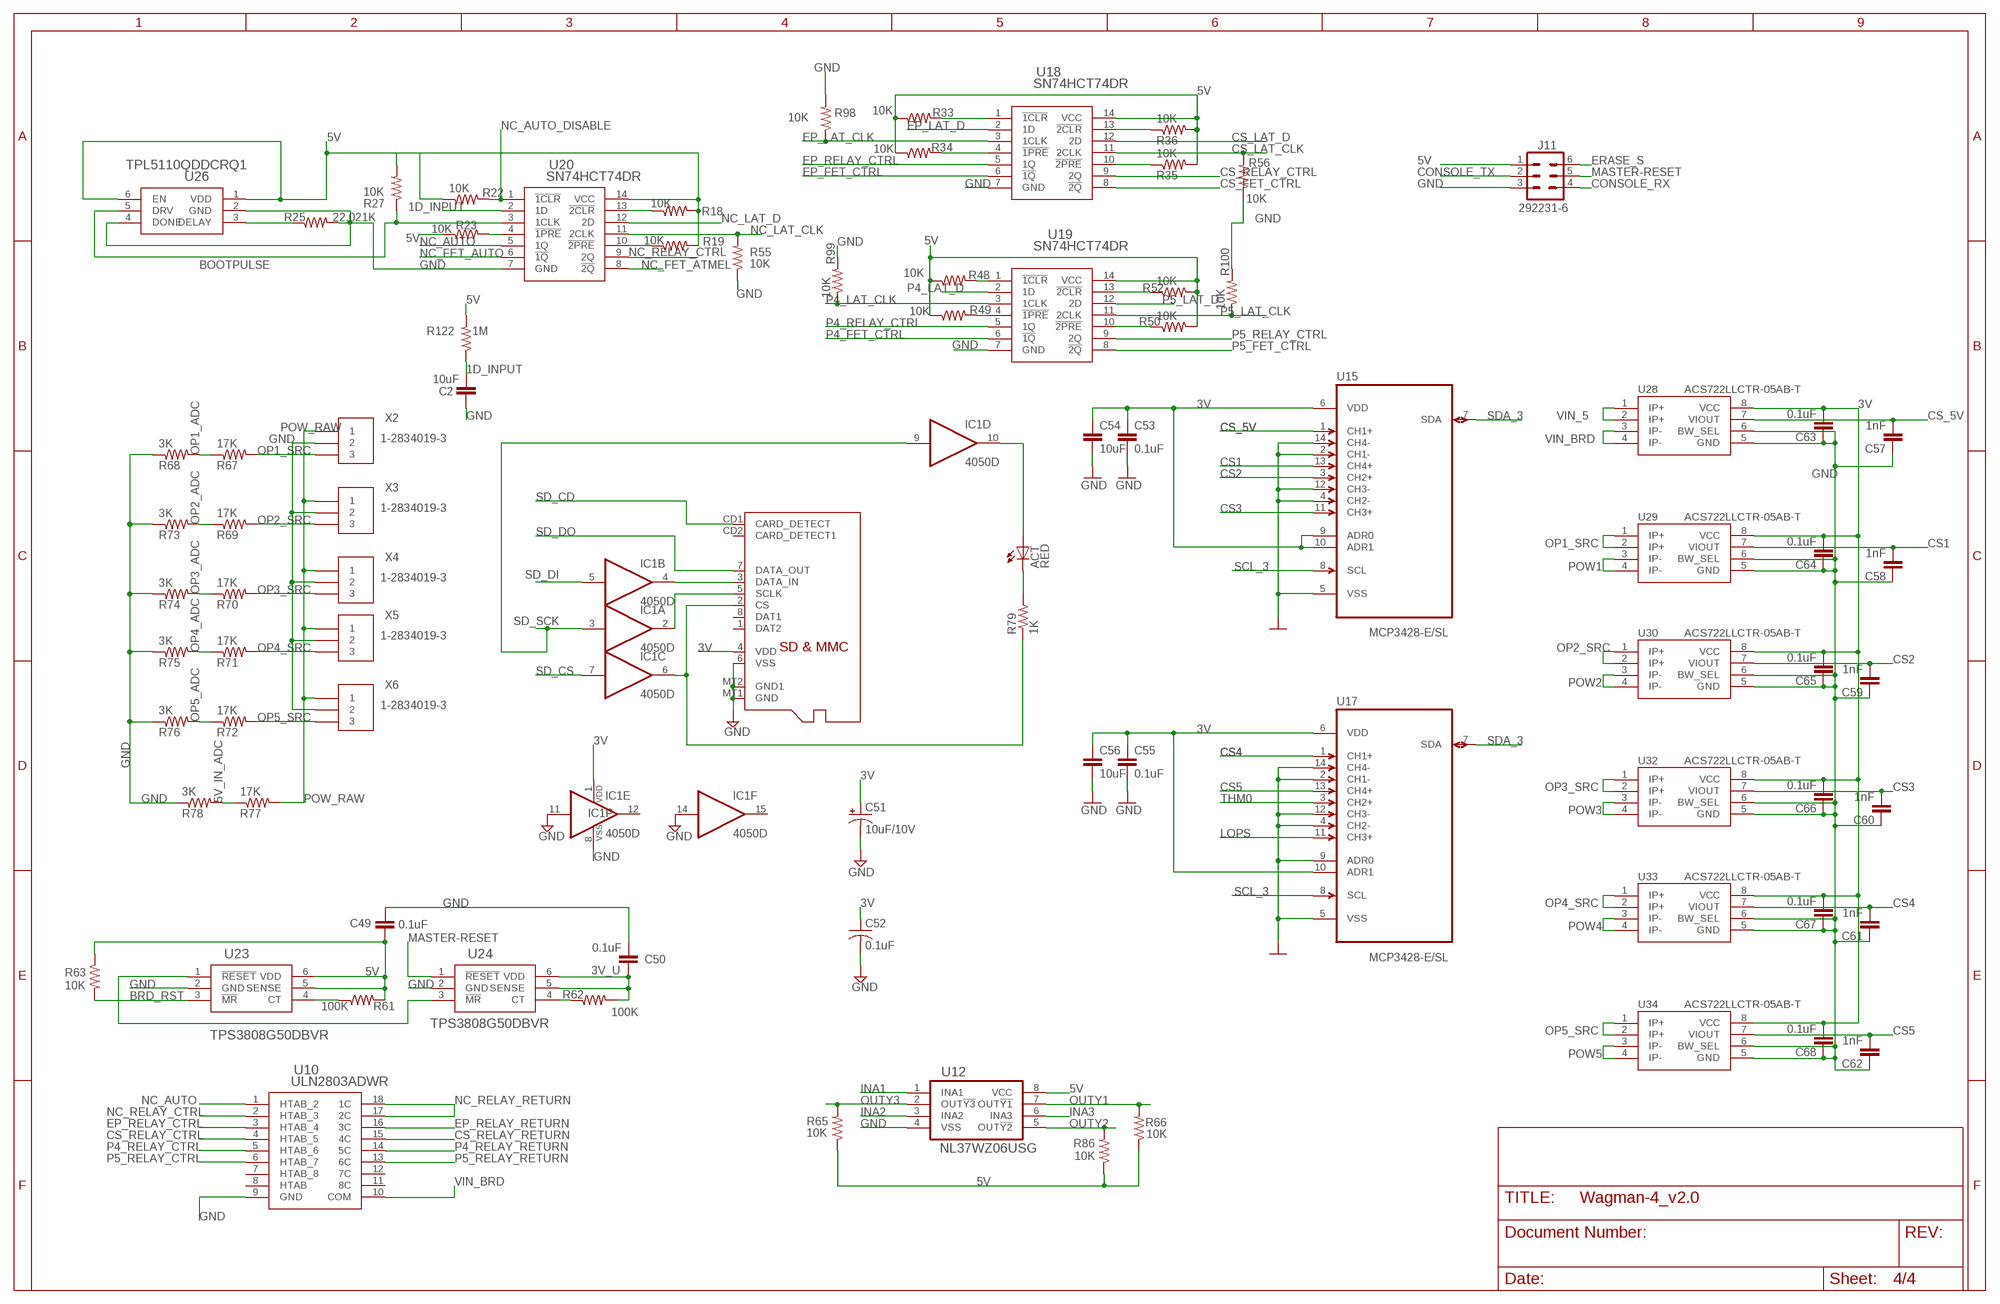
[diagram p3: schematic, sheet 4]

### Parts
ACT  RED  LEDCHIPLED_0805  [CHIPLED_0805]
C2  10uF  CAP0805  [0805]
C49  0.1uF  C-EUC0805  [C0805]
C50  0.1uF  C-EUC0805  [C0805]
C51  10uF/10V  CPOL-USA/3216-18R  [A/3216-18R]
C52  0.1uF  C-USC0805K  [C0805K]
C53  0.1uF  CAP0805  [0805]
C54  10uF  CAP0805  [0805]
C55  0.1uF  CAP0805  [0805]
C56  10uF  CAP0805  [0805]
C57  1nF  CAP0805  [0805]
C58  1nF  CAP0805  [0805]
C59  1nF  CAP0805  [0805]
C60  1nF  CAP0805  [0805]
C61  1nF  CAP0805  [0805]
C62  1nF  CAP0805  [0805]
C63  0.1uF  CAP0805  [0805]
C64  0.1uF  CAP0805  [0805]
C65  0.1uF  CAP0805  [0805]
C66  0.1uF  CAP0805  [0805]
C67  0.1uF  CAP0805  [0805]
C68  0.1uF  CAP0805  [0805]
IC1  4050D  [SO16]
J11  292231-6  [1X6-STRAIGHT-ALT]
R18  10K  R-US_R0805  [R0805]
R19  10K  R-US_R0805  [R0805]
R22  10K  R-US_R0805  [R0805]
R23  10K  R-US_R0805  [R0805]
R25  22.021K  R-US_R0805  [R0805]
R27  10K  R-US_R0805  [R0805]
R33  10K  R-US_R0805  [R0805]
R34  10K  R-US_R0805  [R0805]
R35  10K  R-US_R0805  [R0805]
R36  10K  R-US_R0805  [R0805]
R48  10K  R-US_R0805  [R0805]
R49  10K  R-US_R0805  [R0805]
R50  10K  R-US_R0805  [R0805]
R52  10K  R-US_R0805  [R0805]
R55  10K  R-US_R0805  [R0805]
R56  10K  R-US_R0805  [R0805]
R61  100K  R-US_R0805  [R0805]
R62  100K  R-US_R0805  [R0805]
R63  10K  R-US_R0805  [R0805]
R65  10K  R-US_R0805  [R0805]
R66  10K  R-US_R0805  [R0805]
R67  17K  R-US_R0805  [R0805]
R68  3K  R-US_R0805  [R0805]
R69  17K  R-US_R0805  [R0805]
R70  17K  R-US_R0805  [R0805]
R71  17K  R-US_R0805  [R0805]
R72  17K  R-US_R0805  [R0805]
R73  3K  R-US_R0805  [R0805]
R74  3K  R-US_R0805  [R0805]
R75  3K  R-US_R0805  [R0805]
R76  3K  R-US_R0805  [R0805]
R77  17K  R-US_R0805  [R0805]
R78  3K  R-US_R0805  [R0805]
R79  1K  R-US_R0805  [R0805]
R86  10K  R-US_R0805  [R0805]
R98  10K  R-US_R0805  [R0805]
R99  10K  R-US_R0805  [R0805]
R100  10K  R-US_R0805  [R0805]
R122  1M  R-US_R0805  [R0805]
U10  ULN2803ADWR  [DW18]
U12  NL37WZ06USG  [US-8]
U15  MCP3428-E/SL  [SOIC127P600X175-14N]
U17  MCP3428-E/SL  [SOIC127P600X175-14N]
U18  SN74HCT74DR  [D14]
U19  SN74HCT74DR  [D14]
U20  SN74HCT74DR  [D14]
U23  TPS3808G50DBVR  [DBV6]
U24  TPS3808G50DBVR  [DBV6]
U26  TPL5110QDDCRQ1  [DDC6]
U28  ACS722LLCTR-05AB-T  [SOIC-8]
U29  ACS722LLCTR-05AB-T  [SOIC-8]
U30  ACS722LLCTR-05AB-T  [SOIC-8]
U32  ACS722LLCTR-05AB-T  [SOIC-8]
U33  ACS722LLCTR-05AB-T  [SOIC-8]
U34  ACS722LLCTR-05AB-T  [SOIC-8]
X2  1-2834019-3  [1-2834019-3]
X3  1-2834019-3  [1-2834019-3]
X4  1-2834019-3  [1-2834019-3]
X5  1-2834019-3  [1-2834019-3]
X6  1-2834019-3  [1-2834019-3]
X7  MICROSD  [MICROSD]

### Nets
1D_INPUT: C2.2 R122.1 U20.2(1D)
3V: C51.+ C52.1 C53.1 C54.1 C55.1 C56.1 C63.2 C64.2 C65.2 C66.2 C67.2 C68.2 IC1.1(P:VDD) U15.6(VDD) U15.9(ADR0) U15.10(ADR1) U17.6(VDD) U17.10(ADR1) U28.8(VCC) U29.8(VCC) U30.8(VCC) U32.8(VCC) U33.8(VCC) U34.8(VCC) X7.4(VDD) ; also sheet 1,2,3
3V_U: C50.1 R62.2 U24.5(SENSE) U24.6(VDD) ; also sheet 1,2,3
5V: C49.1 J11.1 R18.2 R19.2 R22.1 R23.1 R27.2 R33.1 R34.1 R35.2 R36.2 R48.1 R49.1 R50.2 R52.2 R61.2 R63.1 R65.1 R66.1 R86.1 R122.2 U12.8(VCC) U18.14(VCC) U19.14(VCC) U20.14(VCC) U23.5(SENSE) U23.6(VDD) U26.1(VDD) U26.6(EN) ; also sheet 1,2,3
5V_IN_ADC: R77.1 R78.2 ; also sheet 1
BOOTPULSE: R27.1 U20.3(1CLK) U26.5(DRV)
BRD_RST: R63.2 U23.3(!MR)
CONSOLE_RX: J11.4 ; also sheet 1
CONSOLE_TX: J11.2 ; also sheet 1
CS1: C58.2 U15.13(CH4+) U29.7(VIOUT)
CS2: C59.2 U15.3(CH2+) U30.7(VIOUT)
CS3: C60.2 U15.11(CH3+) U32.7(VIOUT)
CS4: C61.2 U17.1(CH1+) U33.7(VIOUT)
CS5: C62.2 U17.13(CH4+) U34.7(VIOUT)
CS_5V: C57.2 U15.1(CH1+) U28.7(VIOUT)
CS_FET_CTRL: U18.8(!2Q) ; also sheet 1
CS_LAT_CLK: R56.2 U18.11(2CLK) ; also sheet 1
CS_LAT_D: U18.12(2D) ; also sheet 1
CS_RELAY_CTRL: U10.4(HTAB_5) U18.9(2Q)
CS_RELAY_RETURN: U10.15(4C) ; also sheet 3
EP_FET_CTRL: U18.6(!1Q) ; also sheet 1
EP_LAT_CLK: R98.1 U18.3(1CLK) ; also sheet 1
EP_LAT_D: U18.2(1D) ; also sheet 1
EP_RELAY_CTRL: U10.3(HTAB_4) U18.5(1Q)
EP_RELAY_RETURN: U10.16(3C) ; also sheet 3
ERASE_S: J11.6 ; also sheet 1,2
GND: C2.1 C49.2 C50.2 C51.- C52.2 C53.2 C54.2 C55.2 C56.2 C57.1 C58.1 C59.1 C60.1 C61.1 C62.1 C63.1 C64.1 C65.1 C66.1 C67.1 C68.1 IC1.8(P:VSS) IC1.11(E:I) IC1.14(F:I) J11.3 R25.2 R55.1 R56.1 R68.1 R73.1 R74.1 R75.1 R76.1 R78.1 R98.2 R99.2 R100.2 U10.9(GND) U12.4(VSS) U15.2(CH1-) U15.4(CH2-) U15.5(VSS) U15.12(CH3-) U15.14(CH4-) U17.2(CH1-) U17.4(CH2-) U17.5(VSS) U17.9(ADR0) U17.12(CH3-) U17.14(CH4-) U18.7(GND) U19.7(GND) U20.7(GND) U23.2(GND) U24.2(GND) U26.2(GND) U26.4(DONE) U28.5(GND) U28.6(BW_SEL) U29.5(GND) U29.6(BW_SEL) U30.5(GND) U30.6(BW_SEL) U32.5(GND) U32.6(BW_SEL) U33.5(GND) U33.6(BW_SEL) U34.5(GND) U34.6(BW_SEL) X2.2 X3.2 X4.2 X5.2 X6.2 X7.6(VSS) X7.MT1(GND) X7.MT2(GND1) ; also sheet 1,2,3
INA1: U12.1(INA1) ; also sheet 3
INA2: U12.3(INA2) ; also sheet 3
INA3: U12.6(INA3) ; also sheet 3
LOPS: U17.11(CH3+) ; also sheet 2
MASTER-RESET: J11.5 U24.1(!RESET) ; also sheet 1,2
N$6: R33.2 U18.1(!1CLR)
N$14: R18.1 U20.13(!2CLR)
N$18: R25.1 U26.3(DELAY)
N$20: R19.1 U20.10(!2PRE)
N$24: R23.2 U20.4(!1PRE)
N$28: R34.2 U18.4(!1PRE)
N$30: R35.1 U18.10(!2PRE)
N$45: R36.1 U18.13(!2CLR)
N$46: R48.2 U19.1(!1CLR)
N$47: R49.2 U19.4(!1PRE)
N$48: R50.1 U19.10(!2PRE)
N$49: R52.1 U19.13(!2CLR)
N$58: U23.1(!RESET) U24.3(!MR)
N$59: R61.1 U23.4(CT)
N$60: R62.1 U24.4(CT)
N$63: ACT.A IC1.10(D:O)
N$64: IC1.2(A:O) X7.5(SCLK)
N$65: IC1.6(C:O) R79.1 X7.2(CS)
N$66: ACT.C R79.2
N$67: IC1.4(B:O) X7.3(DATA_IN)
NC_AUTO: U10.1(HTAB_2) U20.5(1Q)
NC_AUTO_DISABLE: R22.2 U20.1(!1CLR) ; also sheet 1
NC_FET_ATMEL: U20.8(!2Q) ; also sheet 2
NC_FET_AUTO: U20.6(!1Q) ; also sheet 2
NC_LAT_CLK: R55.2 U20.11(2CLK) ; also sheet 1
NC_LAT_D: U20.12(2D) ; also sheet 1
NC_RELAY_CTRL: U10.2(HTAB_3) U20.9(2Q)
NC_RELAY_RETURN: U10.17(2C) U10.18(1C) ; also sheet 3
OP1_ADC: R67.1 R68.2 ; also sheet 1
OP1_SRC: R67.2 U29.1(IP+) U29.2(IP+) X2.3
OP2_ADC: R69.1 R73.2 ; also sheet 1
OP2_SRC: R69.2 U30.1(IP+) U30.2(IP+) X3.3
OP3_ADC: R70.1 R74.2 ; also sheet 1
OP3_SRC: R70.2 U32.1(IP+) U32.2(IP+) X4.3
OP4_ADC: R71.1 R75.2 ; also sheet 1
OP4_SRC: R71.2 U33.1(IP+) U33.2(IP+) X5.3
OP5_ADC: R72.1 R76.2 ; also sheet 1
OP5_SRC: R72.2 U34.1(IP+) U34.2(IP+) X6.3
OUTY1: R66.2 U12.7(OUT!Y1) ; also sheet 3
OUTY2: R86.2 U12.5(OUT!Y2) ; also sheet 3
OUTY3: R65.2 U12.2(OUT!Y3) ; also sheet 3
P4_FET_CTRL: U19.6(!1Q) ; also sheet 1
P4_LAT_CLK: R99.1 U19.3(1CLK) ; also sheet 1
P4_LAT_D: U19.2(1D) ; also sheet 1
P4_RELAY_CTRL: U10.5(HTAB_6) U19.5(1Q)
P4_RELAY_RETURN: U10.14(5C) ; also sheet 3
P5_FET_CTRL: U19.8(!2Q) ; also sheet 1
P5_LAT_CLK: R100.1 U19.11(2CLK) ; also sheet 1
P5_LAT_D: U19.12(2D) ; also sheet 1
P5_RELAY_CTRL: U10.6(HTAB_7) U19.9(2Q)
P5_RELAY_RETURN: U10.13(6C) ; also sheet 3
POW1: U29.3(IP-) U29.4(IP-) ; also sheet 1,3
POW2: U30.3(IP-) U30.4(IP-) ; also sheet 1,3
POW3: U32.3(IP-) U32.4(IP-) ; also sheet 1,3
POW4: U33.3(IP-) U33.4(IP-) ; also sheet 1,3
POW5: U34.3(IP-) U34.4(IP-) ; also sheet 1,3
POW_RAW: R77.2 X2.1 X3.1 X4.1 X5.1 X6.1 ; also sheet 3
SCL_3: U15.8(SCL) U17.8(SCL) ; also sheet 1,2,3
SD_CD: X7.CD1(CARD_DETECT) ; also sheet 1
SD_CS: IC1.7(C:I) ; also sheet 1
SD_DI: IC1.5(B:I) ; also sheet 1
SD_DO: X7.7(DATA_OUT) ; also sheet 1
SD_SCK: IC1.3(A:I) IC1.9(D:I) ; also sheet 1
SDA_3: U15.7(SDA) U17.7(SDA) ; also sheet 1,2,3
THM0: U17.3(CH2+) ; also sheet 2
VIN_5: U28.1(IP+) U28.2(IP+) ; also sheet 3
VIN_BRD: U10.10(COM) U28.3(IP-) U28.4(IP-) ; also sheet 1,3
Unconnected: IC1.12(E:O) IC1.15(F:O) U10.11(8C) U10.12(7C) X7.1(DAT2) X7.8(DAT1) X7.CD2(CARD_DETECT1)

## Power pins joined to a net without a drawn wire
HTAB: U10.8(HTAB)
HTAB_8: U10.7(HTAB_8)

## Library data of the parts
ACT L L4 L7-L13 ON ON1 RX TX TX1 = Wagman-4_v1.0:LED: LED
B2 = _jc:COIN-CELL
BR1 = bibaja:J: Three terminal jumper made from two 0402, 0603, 0805, etc.
C1 C3 C43 C45-C50 = resistor:C-EU: CAPACITOR, European symbol
C2 C29 C53-C68 = SparkFun:CAP: Capacitor
C6 C8 C36 C37 C39 = mainBoard_V1R1:CPOL-EU: POLARIZED CAPACITOR, European symbol
C7 C9 C12 C16-C28 C32-C35 C38 C40 C41 C44 = mainBoard:CAP: Capacitor
C11 C13-C15 = _jc:C-US: CAPACITOR, American symbol
C30 PC1-PC3 PC5 = rcl:CPOL-EU: POLARIZED CAPACITOR, European symbol
C31 C42 = wagman_v2.3:CAP: Capacitor
C51 = adafruit:CPOL-US: POLARIZED CAPACITOR, American symbol
C52 = adafruit:C-US: CAPACITOR, American symbol
D1 D6 = Wagman:DIODE: Diode
D3 = _jc:DIODE
D4 = Wagman:DIODE: Diode; PROD_ID: DIO-09646; VALUE: 250mA/100V
EERST ERASE RST = VS_Switches:PTS65SM43SMTR92LFS
F1 = mainBoard_V1R1:L-EU: INDUCTOR, European symbol
F2 = rcl:L-EU: INDUCTOR, European symbol
FD1-FD6 VRF = touch+:FIDUCIAL-1MM
IC1 = 40xx:4050: Hex non-inverting BUFFER
J1 = Wagman-4_v1.0:MC74VHC1G09DTT1G
J2 = Wagman-4_v1.0:022232051
J3 = wagmanV2.2:1051330011_MINIUSB
J4 = VS_Eagle:PXC_277-2066-1-ND
J5-J9 = VS_Eagle:PXC-277-2076-1-ND
J10 = Argon:TB2-3.5MM
J11 = 292231-6:292231-6
JP2 JP3 JP9 = VS_Eagle:CONN_2PIN
JR1 R1 R3-R13 R26 R29 R41 R64 R80 R95 R96 R113-R120 = mainBoard:RESISTOR: Resistor
JTAG = mainBoard_V1R1:PINHEAD_PINHD-2X5: PIN HEADER
K1-K5 = relay:G5LE: RELAY 1 x switch, 10 A/120 V AC, 8 A/30 V DC, Omron; OC_FARNELL: unknown; OC_NEWARK: unknown
L1-L3 L5 L6 = wuerth-elektronik:WE-CBF: SMD EMI Suppression Ferrite Beads
MH1-MH8 = mainBoard:MH-3.964
Q1-Q5 Q8 = SparkFun:MOSFET-NCHANNEL
R2 R14 R15 R37 R88-R94 = SmartPrj:R-EU_: RESISTOR, European symbol
R16 = SparkFun-Sensors:PHOTOCELL: CdS photoresistor. This is a low cost way to detect light levels. Resistance decreases with more incoming light. SparkFun SKU: SEN-09088
R17 R31 R32 R81-R85 R87 R97 R106 R107 R121 = Bourns_By_element14_Batch_1:CRM0805-FW-R050ELF: Resistor 0805; MPN: CRM0805-FW-R050ELF; OC_FARNELL: 1865234; OC_NEWARK: 17T4231; SUPPLIER: BOURNS; TOLERANCE: ±1 %; VALUE: 0.05 Ohm; WATTAGE: 0.25 W
R18 R19 R22 R23 R25 R27 R28 R33-R36 R48-R50 R52-R63 R65-R78 R86 R98-R105 R108-R112 R122 = rcl:R-US_: RESISTOR, American symbol
R20 R21 = _jc:R-US_: RESISTOR, American symbol
R24 R38-R40 R42-R47 = Wagman:PTC-SMD
R30 = wagman_v2.3:CRM0805-FW-R050ELF: Resistor 0805
R51 = Wagman:R-US_: RESISTOR, American symbol
R79 = adafruit:R-US_: RESISTOR, American symbol
RN1 RN3 = mainBoard_V1R1:4R-N: Array Chip Resistor Source: RS Component / Phycomp; OC_FARNELL: unknown; OC_NEWARK: unknown
RN2 = wagman_v2.3:4R-N: Array Chip Resistor Source: RS Component / Phycomp
SJ1-SJ16 = Lightsense_v2.2:SOLDERJUMPER_2WAY: Solder Jumper 2 way solder jumper
SV1 = con-lstb:MA03-2: PIN HEADER; OC_FARNELL: unknown; OC_NEWARK: unknown
SWS001-SWS003 = Argon:CAT872
U1 = mainBoard_V1R1:ATSAM3X/A
U2 = _jc:MCP7941X
U3 U6-U9 U16 U41 = Wagman-4_v1.0:SIS413DN: MOSFET
U4 = Airsense_V3_12-19-2015:24LC256T-E/SN
U5 = Wagman-4_V0.3:AZ1117EH-3.3TRG1
U10 = ULN2803ADWR:ULN2803ADWR; MANUFACTURER_PART_NUMBER: ULN2803ADWR; VENDOR: Texas Instruments
U11 = SysMon:HTU21D
U12 = Wagman-4_v1.0:NL37WZ06USG
U13 U14 U36 U38 U39 = VS_Eagle:CPC1125N
U15 U17 = aux_board_v1r1:MCP3428-E/SL: Analog-to-Digital Converter; MPN: MCP3428-E/SL; OC_FARNELL: 1825014; OC_NEWARK: 52R9962; PACKAGE: SOIC-14; SUPPLIER: Microchip
U18-U20 = SN74HCT74DR:SN74HCT74DR; MANUFACTURER_PART_NUMBER: SN74HCT74DR; VENDOR: Vendor
U21 U22 = Wagman-4_v1.0:TXS0108EPWR; MANUFACTURER_PART_NUMBER: TXS0108EPWR; VENDOR: Texas Instruments
U23 U24 = TPS3808G50DBVR:TPS3808G50DBVR; MANUFACTURER_PART_NUMBER: TPS3808G50DBVR; VENDOR: Texas Instruments
U25 U37 U40 = MC14541BDR2G:MC14541BDR2G; MANUFACTURER_PART_NUMBER: SN74HCT74DR; VENDOR: Vendor
U26 = TPL5110QDDCRQ1:TPL5110QDDCRQ1; MANUFACTURER_PART_NUMBER: TPS3808G50DBVR; VENDOR: Texas Instruments
U28-U30 U32-U34 = Argon:ACS722LLCTR-05AB-T
U31 = Microchip_By_element14_Batch_1:MCP1700T-1802E/TT: Low Quiescent Current LDO; MPN: MCP1700T-1802E/TT; OC_FARNELL: 1296591; OC_NEWARK: 84R5175; PACKAGE: SOT23-3; SUPPLIER: Microchip
X2-X6 = Argon:1-2834019-3
X7 = adafruit:MICROSD: Micro-SD / Transflash card holder with SPI pinout For the 3M # 2908-05WB-MG and/or 4UCON #19656 push-push type
Y1 = mainBoard_V1R1:CRYSTAL-3.2-2.5
Y2 = mainBoard_V1R1:RESONATOR_EPSON_FC_145
Y3 = _jc:CRYSTAL-CITIZEN-CM2XXC
Z1 Z2 = varistor:VARISTOR: VARISTOR

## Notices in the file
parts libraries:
SparkFun-Sensors: Licensing: Creative Commons ShareAlike 4.0 International - https://creativecommons.org/licenses/by-sa/4.0
